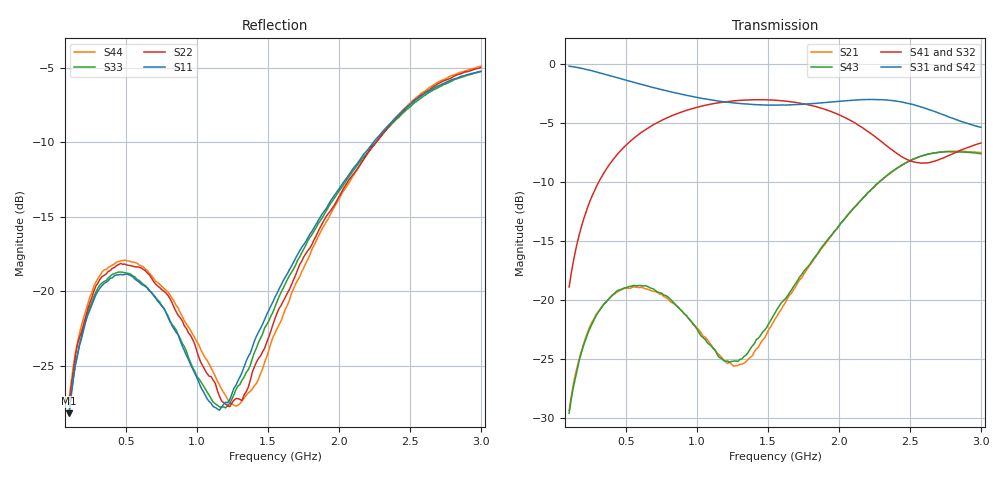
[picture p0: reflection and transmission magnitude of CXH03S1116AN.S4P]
!Agilent Technologies,E5071C,MY46522552,B.13.32
!Date: Tue Dec 24 13:39:28 2024
!Data & Calibration Information:
!Freq	S11:SOLT4(ON)	S12:SOLT4(ON)	S13:SOLT4(ON)	S14:SOLT4(ON)
!	S21:SOLT4(ON)	S22:SOLT4(ON)	S23:SOLT4(ON)	S24:SOLT4(ON)
!	S31:SOLT4(ON)	S32:SOLT4(ON)	S33:SOLT4(ON)	S34:SOLT4(ON)
!	S41:SOLT4(ON)	S42:SOLT4(ON)	S43:SOLT4(ON)	S44:SOLT4(ON)
!PortZ  Port1:50+j0  Port2:50+j0  Port3:50+j0  Port4:50+j0
!Above PortZ is port z conversion or system Z0 setting when saving the data.
!When reading, reference impedance value at option line is always used.
# Hz S dB R 50
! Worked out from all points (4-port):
!   201 points, 100 MHz to 3 GHz, reference 50 ohm
!   strongest paths, dB at 100 MHz, 825 MHz, 1.55 GHz, 2.275 GHz, 3 GHz:
!     S31: -0.1, -2.3, -3.5, -3.0, -5.3
!     S42: -0.1, -2.4, -3.4, -3.0, -5.7
!     S41: -18.9, -4.3, -3.0, -6.3, -6.7
!     S32: -18.9, -4.3, -3.1, -6.3, -6.7
!     S43: -29.6, -20.0, -21.1, -10.1, -7.6
!     S21: -29.3, -20.2, -21.6, -10.1, -7.5
!   lowest |S11| = -28.2 dB at 100 MHz (marker M1), VSWR 1.08, Z = 49.5 - j3.85 ohm
!   |S11| at or under -10 dB: start of sweep to 2.243 GHz
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1e8  -28.20 -94.8  -29.30 72.9  -0.12 -11.0  -18.88 77.7
     -29.33 72.6  -27.53 -96.5  -18.88 77.7  -0.12 -10.8
     -0.14 -11.0  -18.87 77.7  -28.21 -99.9  -29.61 71.7
     -18.87 77.8  -0.14 -10.8  -29.58 71.9  -27.20 -102.3
3.32e8  -19.63 -134.9  -20.51 30.7  -0.75 -34.2  -9.48 53.8
        -20.51 31.0  -19.02 -134.1  -9.47 53.7  -0.75 -33.5
        -0.76 -34.3  -9.47 53.6  -19.45 -136.1  -20.59 27.9
        -9.46 53.7  -0.76 -33.6  -20.55 28.2  -18.71 -135.6
8.25e8  -22.30 162.6  -20.20 -26.7  -2.35 -74.3  -4.35 15.6
        -20.20 -26.7  -20.78 170.1  -4.34 15.2  -2.37 -72.6
        -2.34 -74.4  -4.34 15.2  -22.24 162.5  -20.15 -26.0
        -4.34 15.6  -2.36 -72.6  -20.05 -26.2  -20.48 168.2
1.289e9  -26.02 46.9  -25.52 -15.7  -3.28 -106.0  -3.05 -13.8
         -25.53 -15.1  -27.22 76.9  -3.06 -14.4  -3.29 -103.2
         -3.29 -105.9  -3.07 -14.3  -26.38 50.9  -25.11 -5.9
         -3.05 -13.8  -3.29 -103.2  -25.17 -7.1  -27.65 84.5
2.043e9  -12.55 -32.9  -13.06 -27.3  -3.06 -158.8  -4.50 -57.4
         -13.07 -27.3  -12.95 -27.9  -4.54 -58.1  -3.03 -155.6
         -3.08 -159.0  -4.54 -58.0  -12.72 -35.3  -13.07 -29.5
         -4.50 -57.3  -3.06 -155.8  -13.05 -29.5  -13.13 -29.9
2.5795e9  -6.89 -96.5  -7.78 -90.8  -3.60 151.7  -8.34 -60.1
          -7.77 -91.0  -6.83 -95.5  -8.30 -61.4  -3.73 154.5
          -3.60 151.7  -8.30 -61.4  -7.03 -98.9  -7.76 -91.4
          -8.36 -60.4  -3.71 154.4  -7.76 -91.6  -6.70 -94.9
3e9  -5.22 -142.7  -7.48 -140.3  -5.31 121.3  -6.63 -60.3
     -7.48 -140.1  -4.97 -142.1  -6.71 -62.2  -5.67 124.4
     -5.33 121.4  -6.72 -62.2  -5.24 -144.3  -7.58 -140.6
     -6.66 -60.3  -5.68 124.3  -7.56 -140.6  -4.88 -139.7
